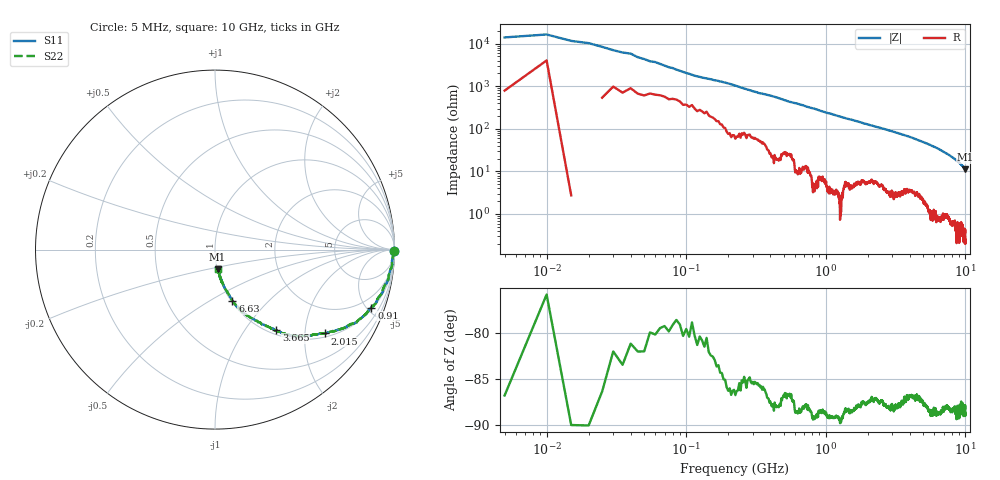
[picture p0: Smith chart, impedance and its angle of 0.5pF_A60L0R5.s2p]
! Amotech Co.,Ltd.
! http://www.amotech.co.kr/
! Part Number: A60L0R5
! These Parameters are Measured in Series Mode Connection
! Operation Temp=25[degC], DC Bias Voltage=0[V]
! Freq. Start=5[MHz] Stop=10[GHz], 2000[Steps]
! Date: Monday, July 14, 2020, 09:25:51
# GHZ S RI R 50.000000
!Freq.(Hz) S11(Real) S11(Imag) S21(Real) S21(Imag) S12(Real) S12(Imag) S22(Real) S22(Imag)
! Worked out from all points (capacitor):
!   2000 points, 5 MHz to 10 GHz, reference 50 ohm
!   read as one part in series: C = 771 fF near 55 MHz
!   lowest |Z| = 11.2 ohm at 9.995 GHz (marker M1)
!   S11 on the Smith chart (normalised r, x): 5 MHz: open; 910 MHz: 1.13, -5.35; 2.015 GHz: 1.11, -2.52; 3.665 GHz: 1.08, -1.42; 6.63 GHz: 1.01, -0.64; 10 GHz: 1.01, -0.23
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0.005  0.9995 -0.00713  0.000454 0.00713  0.000454 0.00713  0.9995 -0.00713
0.035  0.9979 -0.016  0.0021 0.016  0.0021 0.016  0.9979 -0.016
0.08  0.9916 -0.0362  0.00836 0.0362  0.00836 0.0362  0.9916 -0.0362
0.11  0.987 -0.0514  0.013 0.0514  0.013 0.0514  0.987 -0.0514
0.16  0.9861 -0.0704  0.0139 0.0704  0.0139 0.0704  0.9861 -0.0704
0.255  0.9794 -0.1071  0.0206 0.1071  0.0206 0.1071  0.9794 -0.1071
0.345  0.9687 -0.1412  0.0313 0.1412  0.0313 0.1412  0.9687 -0.1412
0.545  0.9386 -0.2134  0.0614 0.2134  0.0614 0.2134  0.9386 -0.2134
0.75  0.9053 -0.2788  0.0947 0.2788  0.0947 0.2788  0.9053 -0.2788
0.91  0.8718 -0.3226  0.1282 0.3226  0.1282 0.3226  0.8718 -0.3226
1.25  0.7902 -0.4011  0.2098 0.4011  0.2098 0.4011  0.7902 -0.4011
1.675  0.6843 -0.4472  0.3157 0.4472  0.3157 0.4472  0.6843 -0.4472
2.015  0.6102 -0.4669  0.3898 0.4669  0.3898 0.4669  0.6102 -0.4669
2.885  0.4518 -0.4832  0.5482 0.4832  0.5482 0.4832  0.4518 -0.4832
3.34  0.3815 -0.4659  0.6185 0.4659  0.6185 0.4659  0.3815 -0.4659
3.665  0.3424 -0.4481  0.6576 0.4481  0.6576 0.4481  0.3424 -0.4481
5.005  0.2006 -0.3806  0.7994 0.3806  0.7994 0.3806  0.2006 -0.3806
6.63  0.0973 -0.2854  0.9027 0.2854  0.9027 0.2854  0.0973 -0.2854
6.67  0.0963 -0.2831  0.9037 0.2831  0.9037 0.2831  0.0963 -0.2831
8.335  0.0432 -0.1901  0.9568 0.1901  0.9568 0.1901  0.0432 -0.1901
9.995  0.0143 -0.11  0.9857 0.11  0.9857 0.11  0.0143 -0.11
10  0.0149 -0.1106  0.9851 0.1106  0.9851 0.1106  0.0149 -0.1106
